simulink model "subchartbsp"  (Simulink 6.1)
settings: Solver=ode1  StartTime=0.0  StopTime=100  FixedStep=0.0001  RelTol=1e-3
libraries: simulink x4

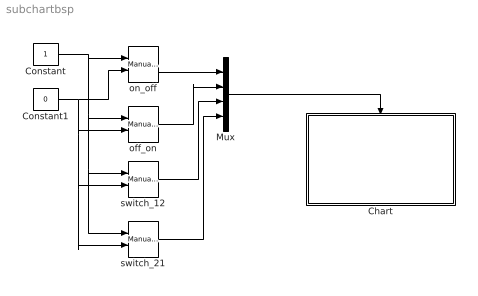
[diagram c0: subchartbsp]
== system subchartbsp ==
  Chart : Stateflow chart  TreatAsAtomicUnit=on
  Constant : Constant
  Constant1 : Constant  Value=0
  Mux : Mux
  off_on : simulink/Signal Routing/Manual Switch  sw=0  action=0
  on_off : simulink/Signal Routing/Manual Switch  sw=0  action=0
  switch_12 : simulink/Signal Routing/Manual Switch  sw=0  action=0
  switch_21 : simulink/Signal Routing/Manual Switch  sw=0  action=0
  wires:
  Constant1/1 -> on_off/2, off_on/2, switch_12/2, switch_21/2
  Constant/1 -> on_off/1, off_on/1, switch_12/1, switch_21/1
  on_off/1 -> Mux/1
  off_on/1 -> Mux/2
  switch_12/1 -> Mux/3
  switch_21/1 -> Mux/4
  Mux/1 -> Chart/Trigger

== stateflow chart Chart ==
  state Z1
    state On
    state Off
    On -> Off : on_off
    Off -> On : off_on
    (default) -> On
  state Z2
    state On
    state Off
    On -> Off : on_off
    Off -> On : off_on
    (default) -> Off
  Z1 -> Z2 : switch_12
  Z2 -> Z1 : switch_21
  (default) -> Z1
